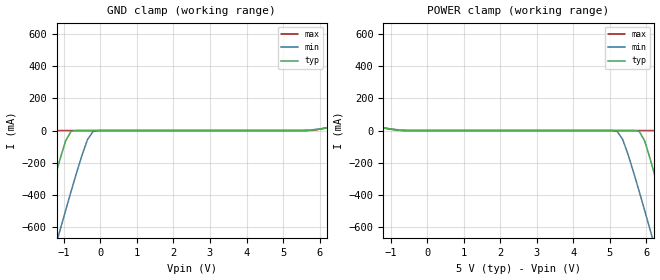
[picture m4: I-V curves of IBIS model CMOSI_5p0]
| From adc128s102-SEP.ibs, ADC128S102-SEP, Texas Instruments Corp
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|   Model CMOSI_5p0
[Model]  CMOSI_5p0
Model_type Input
Polarity   Non-Inverting
Vinl = 0
Vinh = 5.0
C_comp   131.2fF   130.5fF   132fF
[Temperature Range]   25.000   105.00   -40.000
[Voltage Range]   5.0V   4.50V   5.50V
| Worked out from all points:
|   GND clamp passes 1 mA (typ) near -0.68 V on its own axis
|   POWER clamp passes 1 mA (typ) near -0.70 V on its own axis
[Power Clamp]
|Voltage   I(typ)   I(min)   I(max)
-5V       1.94A      1.81A      2.11A
-2.9V     700mA      719mA      687mA
-2.75V    613mA      643mA      587mA
-1.85V    104mA      193mA      48.7mA
-1.1V     12.7mA     12.6mA     12.7mA
5.2V      -13.2pA    -5.65mA    -9.65pA
5.8V      -4.3mA     -376mA     -12.2pA
6.1V      -174mA     -615mA     -8.85nA
6.4V      -423mA     -857mA     -5.69mA
6.7V      -684mA     -1.1A      -215mA
7.15V     -1.08A     -1.47A     -630mA
10V       -3.64A     -3.85A     -3.37A
[Gnd Clamp]
|Voltage   I(typ)   I(min)   I(max)
-5V       -3.64A     -3.85A     -3.37A
-2.15V    -1.08A     -1.47A     -630mA
-1.7V     -684mA     -1.1A      -215mA
-1.4V     -423mA     -857mA     -5.69mA
-1.1V     -174mA     -615mA     -8.85nA
-800mV    -4.3mA     -376mA     -12.2pA
-200mV    -13.2pA    -5.65mA    -9.65pA
6.1V      12.7mA     12.6mA     12.7mA
6.85V     104mA      193mA      48.7mA
7.75V     613mA      643mA      587mA
7.9V      700mA      719mA      687mA
10V       1.94A      1.81A      2.11A
